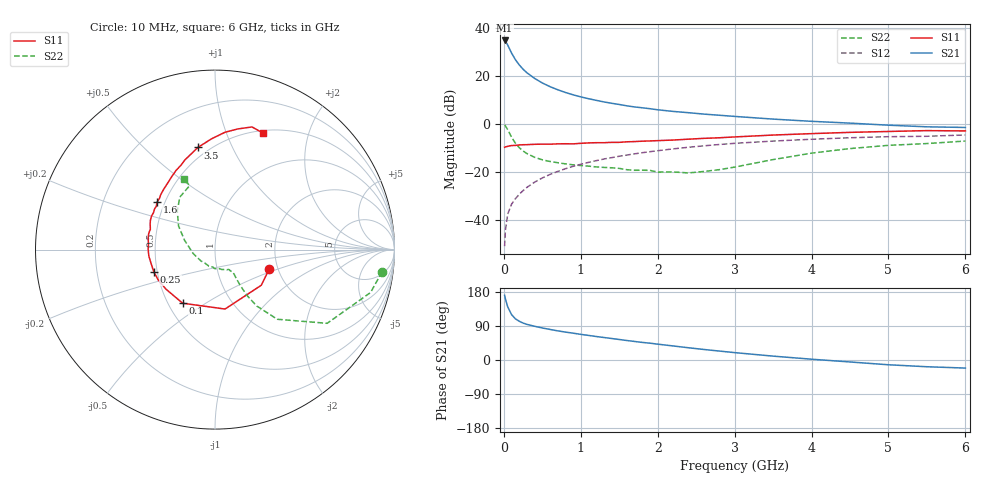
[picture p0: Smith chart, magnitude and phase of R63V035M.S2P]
! SIEMENS Small Signal Semiconductors
! BFR193
! Si NPN RF Bipolar Junction Transistor in SOT23
! VCE = 3 V  IC = 35 mA
! Common Emitter S-Parameters:  May  1996
# GHz  S  MA  R  50
!  f  S11  S21  S12  S22
! GHz  MAG  ANG  MAG  ANG  MAG  ANG  MAG  ANG
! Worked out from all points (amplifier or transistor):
!   36 points, 10 MHz to 6 GHz, reference 50 ohm
!   highest |S21| = 34.6 dB at 10 MHz (marker M1)
!   |S21| within 3 dB of that: start of sweep to 66.57 MHz
!   unconditionally stable (mu >= 1): 456.7 MHz to 1.83 GHz; 1.995148 GHz to 2.002425 GHz
!   at 250 MHz: K = 0.92, MSG = 25.3 dB, |S12| = -27.9 dB
!   at 1.4 GHz: K = 1.02, MAG = 10.5 dB, |S12| = -14.2 dB
!   at 6 GHz: K = 0.95, MSG = 1.6 dB, |S12| = -4.7 dB
!   S11 on the Smith chart (normalised r, x): 10 MHz: 1.80, -0.43; 100 MHz: 0.59, -0.40; 250 MHz: 0.48, -0.14; 1.6 GHz: 0.45, +0.29; 3.5 GHz: 0.44, +0.75; 6 GHz: 0.53, +1.35
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0.01  0.3212 -19.4  53.79 170.6  0.0028 84.3  0.9389 -7.6
0.02  0.3255 -37.6  52.01 161.6  0.0059 82.9  0.8993 -15.4
0.05  0.3358 -80.4  43.24 140.4  0.013 70.7  0.7481 -33.3
0.1  0.3489 -121.1  29.48 119.9  0.0209 65.9  0.5207 -48.2
0.15  0.3508 -140.9  21.46 108.7  0.0272 67.8  0.3909 -53.5
0.2  0.3588 -152.2  16.69 102.3  0.0336 69.4  0.3153 -55.0
0.25  0.3628 -160.0  13.53 97.5  0.0402 70.7  0.2685 -55.0
0.3  0.3636 -166.0  11.43 94.0  0.0469 72.0  0.2379 -54.7
0.4  0.3702 -174.3  8.721 89.0  0.0603 72.8  0.1985 -53.6
0.5  0.3727 179.6  7.009 84.5  0.0737 73.0  0.1758 -52.3
0.6  0.372 175.2  5.875 80.7  0.0873 72.6  0.1626 -52.0
0.7  0.3783 170.1  5.066 76.9  0.1006 71.9  0.1531 -52.8
0.8  0.3801 166.2  4.446 73.7  0.1147 70.7  0.145 -54.4
0.9  0.3778 162.4  3.972 70.8  0.1286 69.8  0.1382 -54.4
1.1  0.3954 155.5  3.298 64.9  0.1554 67.5  0.13 -59.7
1.3  0.3997 149.0  2.827 59.4  0.1827 64.8  0.1223 -64.3
1.6  0.4175 140.4  2.34 51.4  0.2212 60.6  0.1094 -76.4
2.2  0.454 125.7  1.792 37.1  0.2972 51.8  0.0984 -109.9
3.5  0.5769 99.5  1.239 10.2  0.4321 31.5  0.1779 162.8
4.5  0.6562 85.1  1.022 -5.2  0.5068 17.3  0.3016 134.2
5.5  0.7137 73.2  0.856 -17.8  0.5436 3.4  0.3836 111.6
6  0.7025 67.8  0.83 -21.3  0.579 -0.6  0.4328 113.8
